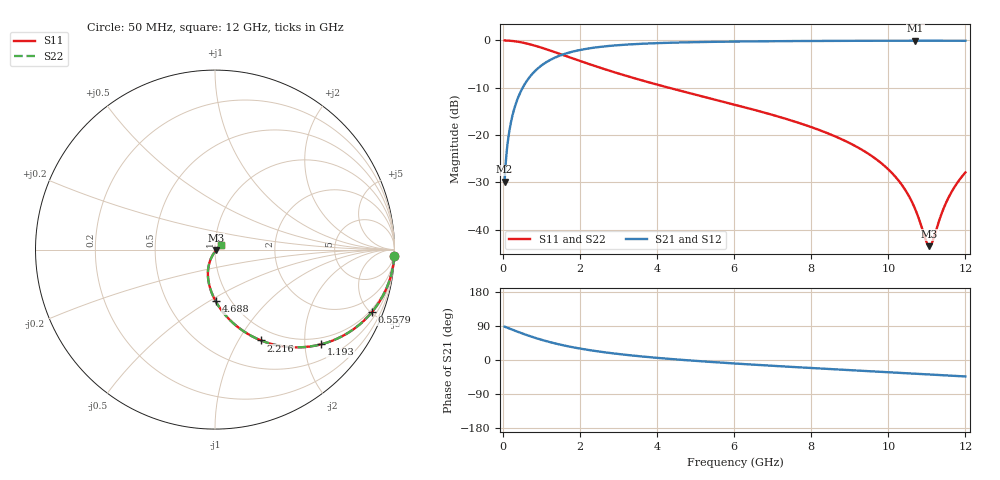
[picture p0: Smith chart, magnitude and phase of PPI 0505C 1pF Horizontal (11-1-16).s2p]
# MHz S MA R 50
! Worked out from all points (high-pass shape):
!   1601 points, 50 MHz to 12 GHz, reference 50 ohm
!   highest |S21| = -0.06 dB at 10.7 GHz (marker M1); lowest = -29.9 dB at 50 MHz (marker M2)
!   |S21| within 3 dB of the highest: 1.53 GHz to end of sweep
!   lowest |S11| = -43.5 dB at 11.07 GHz (marker M3), VSWR 1.01, Z = 50.5 - j0.426 ohm
!   |S11| at or under -10 dB: 4.309 GHz to end of sweep
!   |S22| runs from -43.5 to 0.0 dB; largest |S21 - S12| = 0
!   S11 on the Smith chart (normalised r, x): 50 MHz: 1, -57; 557.9 MHz: 0.83, -5.08; 1.193 GHz: 0.84, -2.36; 2.216 GHz: 0.84, -1.25; 4.688 GHz: 0.85, -0.54; 12 GHz: 1.07, +0.05
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50  0.9995 -2.0  0.0321 88.0  0.0321 88.0  0.9995 -2.0
154.5625  0.9951 -6.2  0.09879 83.8  0.09879 83.8  0.9951 -6.2
236.7188  0.9886 -9.5  0.1503 80.5  0.1503 80.5  0.9886 -9.5
371.1562  0.9726 -14.7  0.232 75.2  0.232 75.2  0.9726 -14.7
557.875  0.941 -21.7  0.3375 68.2  0.3375 68.2  0.941 -21.7
1192.719  0.7917 -41.8  0.6094 48.1  0.6094 48.1  0.7917 -41.8
2044.156  0.5993 -60.3  0.7982 29.5  0.7982 29.5  0.5993 -60.3
2215.938  0.5671 -63.1  0.8211 26.6  0.8211 26.6  0.5671 -63.1
3022.562  0.4446 -74.0  0.8926 15.6  0.8926 15.6  0.4446 -74.0
4038.312  0.3385 -84.0  0.9373 5.4  0.9373 5.4  0.3385 -84.0
4688.094  0.2881 -89.2  0.9536 0.1  0.9536 0.1  0.2881 -89.2
6025  0.2089 -98.1  0.9733 -9.3  0.9733 -9.3  0.2089 -98.1
8019.156  0.1206 -108.8  0.9871 -21.2  0.9871 -21.2  0.1206 -108.8
9191.75  0.07468 -113.4  0.991 -27.8  0.991 -27.8  0.07468 -113.4
10013.31  0.04286 -114.2  0.9924 -32.3  0.9924 -32.3  0.04286 -114.2
10401.69  0.02777 -111.4  0.9927 -34.5  0.9927 -34.5  0.02777 -111.4
10700.44  0.01638 -102.9  0.9928 -36.1  0.9928 -36.1  0.01638 -102.9
10976.78  0.00764 -67.5  0.9927 -37.7  0.9927 -37.7  0.00764 -67.5
11066.41  0.00668 -39.1  0.9926 -38.2  0.9926 -38.2  0.00668 -39.1
11148.56  0.007485 -12.6  0.9926 -38.6  0.9926 -38.6  0.007485 -12.6
11559.34  0.02168 30.3  0.9921 -40.9  0.9921 -40.9  0.02168 30.3
12000  0.04022 36.2  0.9913 -43.4  0.9913 -43.4  0.04022 36.2
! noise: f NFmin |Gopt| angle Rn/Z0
50  0.001158  0.9695  1.53  0.008613
1372  0.005838  0.7701  7.193  0.005154
2701  0.009186  0.7179  11.47  0.006378
4031  0.01215  0.6878  15.86  0.007421
5360  0.01493  0.6681  20.25  0.008383
6682  0.01762  0.6551  24.55  0.009317
8012  0.02032  0.647  28.81  0.01027
9341  0.02306  0.6428  32.96  0.01127
1.067e+04  0.02588  0.6419  37.01  0.01235
1.2e+04  0.02883  0.6438  40.94  0.01353
